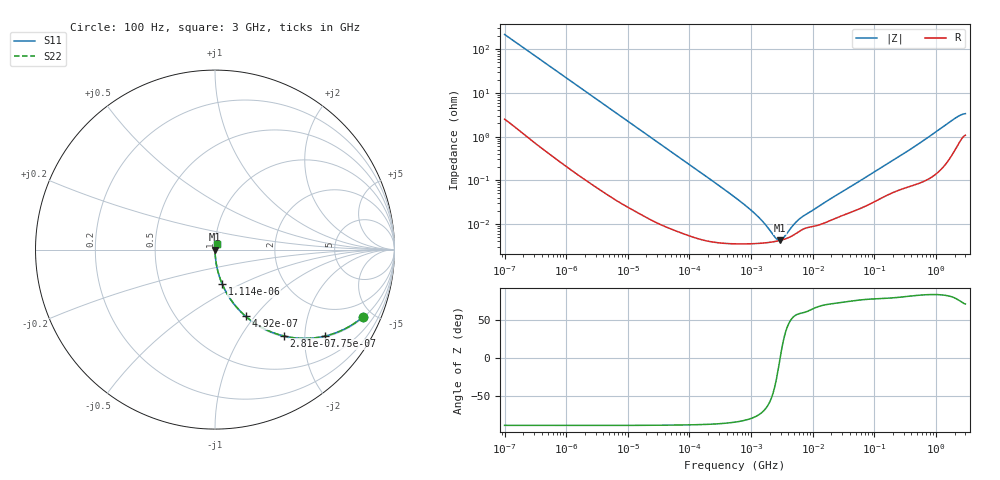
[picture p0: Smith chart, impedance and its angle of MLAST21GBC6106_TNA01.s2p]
! MLAST21GBC6106_TNA01  S-PARAMETER MODEL  ( Standard Model )
! Model Generated by TAIYO YUDEN Corporation (http://www.ty-top.com)
! Version 1.0
! TAIYO YUDEN Control No. 220601
! Copyright(c) 2019 TAIYO YUDEN CO.,LTD. All Rights Reserved.
! Product Description (link to TY-COMPAS)
! https://ds.yuden.co.jp/TYCOMPAS/or/detail?pn=MLAST21GBC6106KTNA01&u=M
! Products Name : Multilayer Ceramic Capacitors
! Characteristics :
!  Capacitance : 10 [uF] , Rated Voltage : 25 [V] , TCC : X6S
!  Case Size : 2.0 x 1.25 / 0.079 x 0.049 [mm/inch] , Thickness : 1.25 / 0.049 [mm/inch]
!  (Conditions: Temperature = 25 [degC] , DC Bias Voltage = 0 [V])
! External Node Assignments :
!  1  o---| |---o  2
! GND o---------o GND
! Frequency Range : 100Hz  -  3GHz  [ 401 STEP ]
# MHZ S RI R 50
! Freq[MHz].  S11 Real  S11 Imag  S21 Real  S21 Imag  S12 Real  S12 Imag  S22 Real  S22 Imag
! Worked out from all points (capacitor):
!   401 points, 100 Hz to 3 GHz, reference 50 ohm
!   read as one part in series: C = 7.26 uF near 109 Hz
!   lowest |Z| = 4.18 mohm at 2.935 MHz (marker M1)
!   series resonance near 2.96 MHz, so ESL is about 400 pH
!   S11 on the Smith chart (normalised r, x): 100 Hz: 1.05, -4.38; 175 Hz: 1.03, -2.51; 281 Hz: 1.02, -1.57; 492 Hz: 1.01, -0.90; 1.114 kHz: 1.00, -0.40; 3 GHz: 1.02, +0.06
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0.0001  0.8245 -0.3747  0.1755 0.3747  0.1755 0.3747  0.8245 -0.3747
0.000119  0.7704 -0.4149  0.2296 0.4149  0.2296 0.4149  0.7704 -0.4149
0.000175  0.611 -0.4821  0.389 0.4821  0.389 0.4821  0.611 -0.4821
0.000281  0.3825 -0.4809  0.6175 0.4809  0.6175 0.4809  0.3825 -0.4809
0.000492  0.1709 -0.3716  0.8291 0.3716  0.8291 0.3716  0.1709 -0.3716
0.000724  0.0879 -0.2785  0.9121 0.2785  0.9121 0.2785  0.0879 -0.2785
0.001114  0.04 -0.1913  0.96 0.1913  0.96 0.1913  0.04 -0.1913
0.001788  0.0164 -0.1225  0.9836 0.1225  0.9836 0.1225  0.0164 -0.1225
0.005476  0.00207 -0.0409  0.9979 0.0409  0.9979 0.0409  0.00207 -0.0409
0.031977  0.00015 -0.00709  0.9998 0.00709  0.9998 0.00709  0.00015 -0.00709
0.547723  3.51e-05 -0.000405  1 0.000405  1 0.000405  3.51e-05 -0.000405
0.958445  3.5e-05 -0.000214  1 0.000214  1 0.000214  3.5e-05 -0.000214
1.677156  3.67e-05 -9.22e-05  1 9.22e-05  1 9.22e-05  3.67e-05 -9.22e-05
2.93481  4.17e-05 -1.3e-06  1 1.3e-06  1 1.3e-06  4.17e-05 -1.3e-06
4.91919  5.58e-05 7.88e-05  0.9999 -7.88e-05  0.9999 -7.88e-05  5.58e-05 7.88e-05
6.941223  7.55e-05 0.000129  0.9999 -0.000129  0.9999 -0.000129  7.55e-05 0.000129
9.794414  8.65e-05 0.000182  0.9999 -0.000182  0.9999 -0.000182  8.65e-05 0.000182
175.1444  0.000486 0.0025  0.9995 -0.0025  0.9995 -0.0025  0.000486 0.0025
492.0662  0.000857 0.00639  0.9991 -0.00639  0.9991 -0.00639  0.000857 0.00639
2036.508  0.00558 0.0255  0.9944 -0.0255  0.9944 -0.0255  0.00558 0.0255
2525.516  0.00914 0.0297  0.9909 -0.0297  0.9909 -0.0297  0.00914 0.0297
3000  0.0116 0.0311  0.9884 -0.0311  0.9884 -0.0311  0.0116 0.0311
